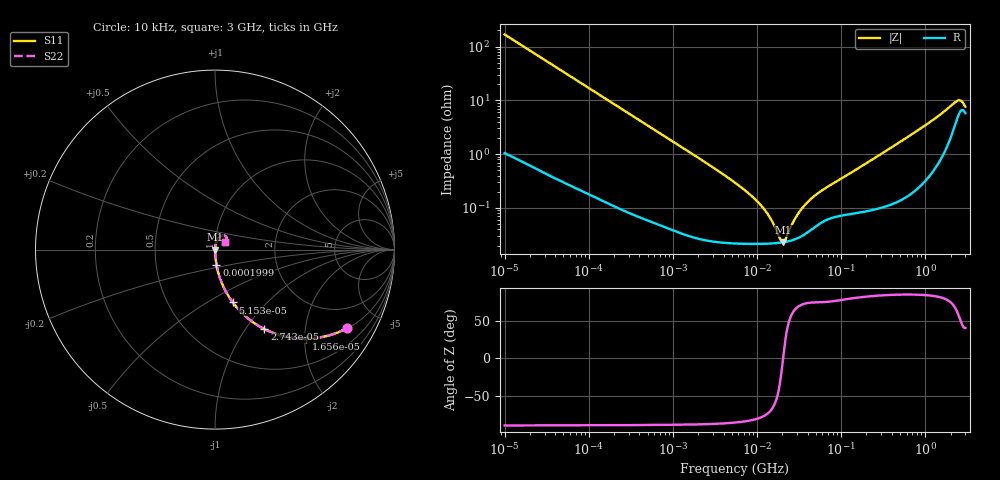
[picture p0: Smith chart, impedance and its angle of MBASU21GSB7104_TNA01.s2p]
! MBASU21GSB7104_TNA01  S-PARAMETER MODEL  ( Standard Model )
! Model Generated by TAIYO YUDEN Corporation (http://www.ty-top.com)
! Version 1.0
! TAIYO YUDEN Control No. 220601
! Copyright(c) 2012 TAIYO YUDEN CO.,LTD. All Rights Reserved.
! Product Description (link to TY-COMPAS)
! https://ds.yuden.co.jp/TYCOMPAS/or/detail?pn=MBASU21GSB7104KTNA01&u=M
! Products Name : Multilayer Ceramic Capacitors
! Characteristics :
!  Capacitance : 0.1 [uF] , Rated Voltage : 50 [V] , TCC : X7R
!  Case Size : 2.0 x 1.25 / 0.079 x 0.049 [mm/inch] , Thickness : 1.25 / 0.049 [mm/inch]
!  (Conditions: Temperature = 25 [degC] , DC Bias Voltage = 0 [V])
! External Node Assignments :
!  1  o---| |---o  2
! GND o---------o GND
! Frequency Range : 10kHz  -  3GHz  [ 401 STEP ]
# MHZ S RI R 50
! Freq[MHz].  S11 Real  S11 Imag  S21 Real  S21 Imag  S12 Real  S12 Imag  S22 Real  S22 Imag
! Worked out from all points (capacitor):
!   401 points, 10 kHz to 3 GHz, reference 50 ohm
!   read as one part in series: C = 94.8 nF near 10.65 kHz
!   lowest |Z| = 23.1 mohm at 20.59 MHz (marker M1)
!   series resonance near 20.41 MHz, so ESL is about 640 pH
!   S11 on the Smith chart (normalised r, x): 10 kHz: 1.02, -3.35; 16.56 kHz: 1.01, -2.03; 27.43 kHz: 1.01, -1.23; 51.53 kHz: 1.01, -0.66; 199.9 kHz: 1.00, -0.17; 3 GHz: 1.12, +0.10
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0.01  0.7365 -0.4374  0.2635 0.4374  0.2635 0.4374  0.7365 -0.4374
0.016561  0.5074 -0.4965  0.4926 0.4965  0.4926 0.4965  0.5074 -0.4965
0.027426  0.2755 -0.4429  0.7245 0.4429  0.7245 0.4429  0.2755 -0.4429
0.051526  0.0992 -0.2946  0.9008 0.2946  0.9008 0.2946  0.0992 -0.2946
0.082683  0.0421 -0.1959  0.9579 0.1959  0.9579 0.1959  0.0421 -0.1959
0.199902  0.00826 -0.0844  0.9917 0.0844  0.9917 0.0844  0.00826 -0.0844
0.683653  0.00111 -0.0251  0.9989 0.0251  0.9989 0.0251  0.00111 -0.0251
5.477226  0.000227 -0.00295  0.9998 0.00295  0.9998 0.00295  0.000227 -0.00295
8.516475  0.000218 -0.00169  0.9998 0.00169  0.9998 0.00169  0.000218 -0.00169
11.67315  0.000217 -0.00101  0.9998 0.00101  0.9998 0.00101  0.000217 -0.00101
14.55585  0.000219 -0.00059  0.9998 0.00059  0.9998 0.00059  0.000219 -0.00059
18.73182  0.000226 -0.000147  0.9998 0.000147  0.9998 0.000147  0.000226 -0.000147
20.5901  0.000231 1.53e-05  0.9998 -1.53e-05  0.9998 -1.53e-05  0.000231 1.53e-05
21.93027  0.000235 0.000124  0.9998 -0.000124  0.9998 -0.000124  0.000235 0.000124
26.49725  0.000253 0.000456  0.9997 -0.000456  0.9997 -0.000456  0.000253 0.000456
31.02164  0.000279 0.000743  0.9997 -0.000743  0.9997 -0.000743  0.000279 0.000743
45.28751  0.000407 0.00149  0.9996 -0.00149  0.9996 -0.00149  0.000407 0.00149
374.4521  0.00128 0.0125  0.9987 -0.0125  0.9987 -0.0125  0.00128 0.0125
1093.834  0.00511 0.0374  0.9949 -0.0374  0.9949 -0.0374  0.00511 0.0374
2331.196  0.0452 0.0793  0.9548 -0.0793  0.9548 -0.0793  0.0452 0.0793
2644.539  0.0647 0.0663  0.9353 -0.0663  0.9353 -0.0663  0.0647 0.0663
3000  0.0567 0.0444  0.9433 -0.0444  0.9433 -0.0444  0.0567 0.0444
